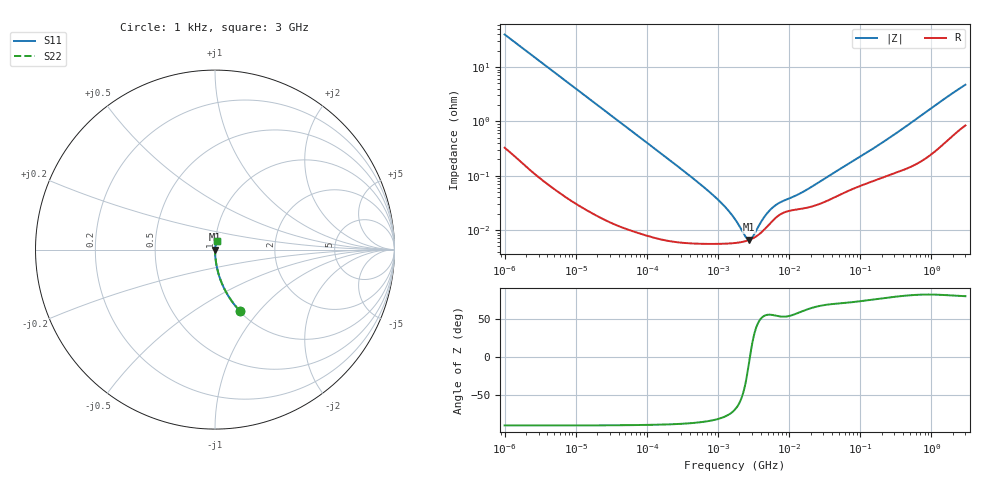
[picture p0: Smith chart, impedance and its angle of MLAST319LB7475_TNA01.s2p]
! MLAST319LB7475_TNA01  S-PARAMETER MODEL  ( Standard Model )
! Model Generated by TAIYO YUDEN Corporation (http://www.ty-top.com)
! Version 1.0
! TAIYO YUDEN Control No. 220601
! Copyright(c) 2011 TAIYO YUDEN CO.,LTD. All Rights Reserved.
! Product Description (link to TY-COMPAS)
! https://ds.yuden.co.jp/TYCOMPAS/or/detail?pn=MLAST319LB7475KTNA01&u=M
! Products Name : Multilayer Ceramic Capacitors
! Characteristics :
!  Capacitance : 4.7 [uF] , Rated Voltage : 25 [V] , TCC : X7R
!  Case Size : 3.2 x 1.6 / 0.126 x 0.063 [mm/inch] , Thickness : 0.85 / 0.033 [mm/inch]
!  (Conditions: Temperature = 25 [degC] , DC Bias Voltage = 0 [V])
! External Node Assignments :
!  1  o---| |---o  2
! GND o---------o GND
! Frequency Range : 1kHz  -  3GHz  [ 401 STEP ]
# MHZ S RI R 50
! Freq[MHz].  S11 Real  S11 Imag  S21 Real  S21 Imag  S12 Real  S12 Imag  S22 Real  S22 Imag
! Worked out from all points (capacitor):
!   401 points, 1 kHz to 3 GHz, reference 50 ohm
!   read as one part in series: C = 4 uF near 1.077 kHz
!   lowest |Z| = 6.61 mohm at 2.709 MHz (marker M1)
!   series resonance near 2.807 MHz, so ESL is about 800 pH
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0.001  0.1383 -0.3411  0.8617 0.3411  0.8617 0.3411  0.1383 -0.3411
0.001685  0.0545 -0.2231  0.9455 0.2231  0.9455 0.2231  0.0545 -0.2231
0.00306  0.0176 -0.1281  0.9824 0.1281  0.9824 0.1281  0.0176 -0.1281
0.005768  0.00528 -0.069  0.9947 0.069  0.9947 0.069  0.00528 -0.069
0.01216  0.00135 -0.033  0.9987 0.033  0.9987 0.033  0.00135 -0.033
0.147855  7.6e-05 -0.00274  0.9999 0.00274  0.9999 0.00274  7.6e-05 -0.00274
0.43594  5.74e-05 -0.000912  0.9999 0.000912  0.9999 0.000912  5.74e-05 -0.000912
0.821683  5.57e-05 -0.000455  0.9999 0.000455  0.9999 0.000455  5.57e-05 -0.000455
1.285341  5.62e-05 -0.000252  0.9999 0.000252  0.9999 0.000252  5.62e-05 -0.000252
1.732051  5.77e-05 -0.000148  0.9999 0.000148  0.9999 0.000148  5.77e-05 -0.000148
2.166294  6.02e-05 -7.76e-05  0.9999 7.76e-05  0.9999 7.76e-05  6.02e-05 -7.76e-05
2.334012  6.15e-05 -5.51e-05  0.9999 5.51e-05  0.9999 5.51e-05  6.15e-05 -5.51e-05
2.709407  6.52e-05 -1.06e-05  0.9999 1.06e-05  0.9999 1.06e-05  6.52e-05 -1.06e-05
3.264662  7.32e-05 4.53e-05  0.9999 -4.53e-05  0.9999 -4.53e-05  7.32e-05 4.53e-05
3.517417  7.79e-05 6.79e-05  0.9999 -6.79e-05  0.9999 -6.79e-05  7.79e-05 6.79e-05
4.919932  0.000117 0.000168  0.9999 -0.000168  0.9999 -0.000168  0.000117 0.000168
6.629817  0.000173 0.000238  0.9998 -0.000238  0.9998 -0.000238  0.000173 0.000238
13.97519  0.000243 0.000397  0.9998 -0.000397  0.9998 -0.000397  0.000243 0.000397
21.06097  0.000272 0.000572  0.9997 -0.000572  0.9997 -0.000572  0.000272 0.000572
256.0921  0.00104 0.00485  0.999 -0.00485  0.999 -0.00485  0.00104 0.00485
1652.1  0.00509 0.0274  0.9949 -0.0274  0.9949 -0.0274  0.00509 0.0274
3000  0.0105 0.0456  0.9895 -0.0456  0.9895 -0.0456  0.0105 0.0456
